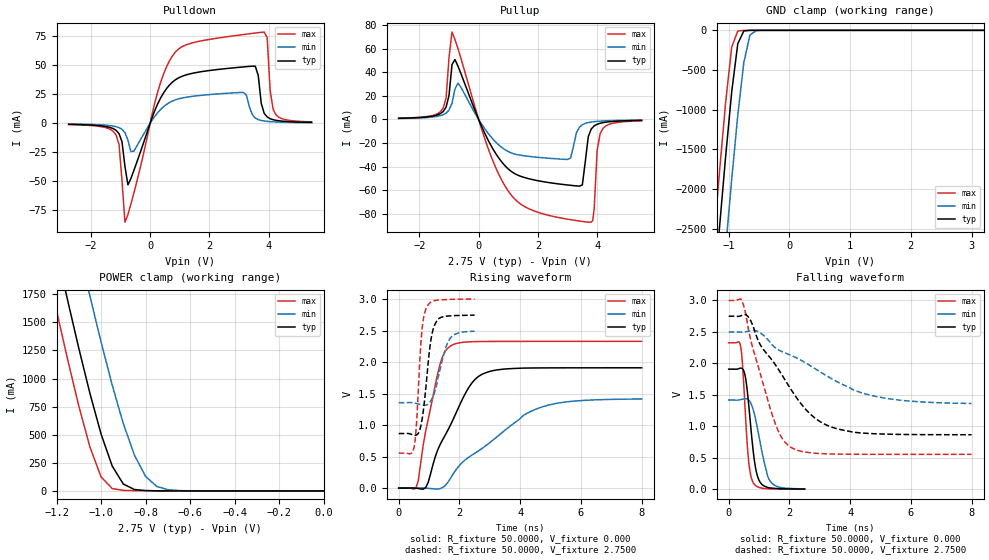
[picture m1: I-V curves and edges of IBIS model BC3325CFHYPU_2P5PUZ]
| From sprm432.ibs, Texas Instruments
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|   Model BC3325CFHYPU_2P5PUZ
[Model]   BC3325CFHYPU_2P5PUZ
Model_type   I/O
Polarity   Non-Inverting
Enable   Active-Low
Vinl =   0.8250V
Vinh =   1.9250V
Vmeas =   1.3750V
Cref =  15.0000pF
Rref = 100.0000M
Vref =  0.000V
C_comp   3.2189pF   3.2468pF   3.2081pF
[Temperature Range]   25.0000   0.1250k   -40.0000
[Voltage Range]   2.7500V   2.5000V   3.0000V
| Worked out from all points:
|   slope of the pulldown table from 0 to 0.412 V, typ, clamps not added: 16.9 ohm
|   slope of the pullup table from 0 to 0.412 V, typ, clamps not added: 18.8 ohm
|   GND clamp passes 1 mA (typ) near -0.66 V on its own axis
|   POWER clamp passes 1 mA (typ) near -0.73 V on its own axis
|   rising waveform, R_fixture 50.0000, V_fixture 0.000: 20-80 % time 1.09ns typ, 2.18ns min, 565ps max; typ from 0.001 V to 1.91 V
|   rising waveform, R_fixture 50.0000, V_fixture 2.7500: 20-80 % time 253ps typ, 352ps min, 179ps max; typ from 0.866 V to 2.74 V
|   falling waveform, R_fixture 50.0000, V_fixture 0.000: 20-80 % time 249ps typ, 370ps min, 182ps max; typ from 1.91 V to 0.003 V
|   falling waveform, R_fixture 50.0000, V_fixture 2.7500: 20-80 % time 1.63ns typ, 2.58ns min, 870ps max; typ from 2.75 V to 0.866 V
[Pulldown]
| voltage   I(typ)   I(min)   I(max)
-2.75V    -942uA     -650uA     -1.139mA
-1.15V    -6.095mA   -2.984mA   -10.11mA
-850mV    -37.32mA   -8.056mA   -85.29mA
-550mV    -40.73mA   -24mA      -60.28mA
350mV     21.58mA    11.77mA    34.97mA
1.05V     40.19mA    21.58mA    65.58mA
3.15V     48.55mA    26.51mA    76.47mA
3.55V     49.14mA    4.498mA    77.79mA
3.85V     8.531mA    1.96mA     78.57mA
3.95V     5.417mA    1.638mA    73.77mA
4.15V     3.05mA     1.228mA    12mA
5.45V     763uA      461uA      1.156mA
[Pullup]
| voltage   I(typ)   I(min)   I(max)
-2.7V     969uA      801uA      1.062mA
-1.2V     6.636mA    4.013mA    9.53mA
-900mV    46.54mA    13.78mA    74.18mA
-700mV    45.39mA    30.78mA    60.33mA
1V        -42.09mA   -27.31mA   -60.87mA
3V        -55.65mA   -33.97mA   -84.69mA
3.4V      -56.64mA   -6.607mA   -86.26mA
3.7V      -14.63mA   -2.671mA   -87.24mA
3.85V     -6.779mA   -2.044mA   -85.88mA
4V        -4.071mA   -1.633mA   -26.15mA
4.1V      -3.234mA   -1.443mA   -12mA
5.5V      -811uA     -542uA     -1.185mA
[GND_clamp]
| voltage   I(typ)   I(min)   I(max)
-2.75V    -17.96A    -19.08A    -17.31A
-1.25V    -3.392A    -4.569A    -2.686A
-1.15V    -2.474A    -3.647A    -1.77A
-1.05V    -1.588A    -2.744A    -906.7mA
-950mV    -773.4mA   -1.875A    -209.9mA
-850mV    -168.6mA   -1.068A    -9.074mA
-750mV    -7.37mA    -403.3mA   -1.005mA
-650mV    -331.2uA   -59.95mA   -203.1uA
-550mV    -99.07uA   -4.004mA   -142.8uA
3.2V      0A         0A         0A
[POWER_clamp]
| voltage   I(typ)   I(min)   I(max)
-2.75V    17.1A      17.93A     16.63A
-1.25V    2.586A     3.492A     2.054A
-1.2V     2.135A     3.04A      1.604A
-1.15V    1.695A     2.594A     1.168A
-1.05V    867.5mA    1.733A     390.4mA
-1V       506.6mA    1.325A     125mA
-950mV    221.5mA    942.3mA    21.02mA
-900mV    61.16mA    598.6mA    4.683mA
-850mV    12.38mA    317.4mA    2.264mA
-800mV    3.105mA    129.1mA    1.319mA
-750mV    1.226mA    39.97mA    719.2uA
0V        226.1pA    1.421nA    243.2pA
[Ramp]
| variable   typ   min   max
dV/dt_r   1.0381/0.9480n   0.3340/0.5367n   1.3934/0.5563n
dV/dt_f   0.8857/1.1637n   0.2933/0.8931n   1.4454/0.8421n
R_load = 50.0000
[Rising Waveform]
R_fixture = 50.0000
V_fixture = 0.000
V_fixture_min = 0.000
V_fixture_max = 0.000
| time   V(typ)   V(min)   V(max)
0s        897uV      859.3uV    954.2uV
565.7ps   -639.9uV   1.934mV    -4.572mV
646.5ps   -5.914mV   1.935mV    121.3mV
888.9ps   8.314mV    -475.1uV   902.6mV
1.293ns   614.7mV    -13.65mV   1.831V
1.697ns   992.8mV    150mV      2.252V
2.424ns   1.675V     527.4mV    2.323V
2.99ns    1.85V      717.4mV    2.327V
4.848ns   1.907V     1.306V     2.328V
8ns       1.909V     1.414V     2.328V
[Rising Waveform]
R_fixture = 50.0000
V_fixture = 2.7500
V_fixture_min = 2.5000
V_fixture_max = 3.0000
| time   V(typ)   V(min)   V(max)
0s        866.2mV    1.355V     555.2mV
505.1ps   839.9mV    1.351V     644.6mV
580.8ps   841mV      1.343V     976.6mV
757.6ps   1.053V     1.321V     2.457V
833.3ps   1.311V     1.315V     2.732V
934.3ps   1.796V     1.323V     2.879V
1.086ns   2.417V     1.407V     2.958V
1.288ns   2.677V     1.735V     2.983V
1.692ns   2.732V     2.373V     2.993V
2.5ns     2.744V     2.488V     2.999V
[Falling Waveform]
R_fixture = 50.0000
V_fixture = 0.000
V_fixture_min = 0.000
V_fixture_max = 0.000
| time   V(typ)   V(min)   V(max)
0s        1.909V     1.417V     2.328V
404ps     1.926V     1.426V     2.244V
454.5ps   1.915V     1.432V     1.991V
530.3ps   1.831V     1.439V     1.376V
631.3ps   1.48V      1.43V      586.2mV
707.1ps   1.098V     1.389V     268.8mV
808.1ps   605.5mV    1.264V     104.5mV
984.8ps   159.3mV    876.3mV    32.88mV
1.364ns   21.51mV    131.5mV    6.622mV
2.5ns     3.408mV    6.945mV    1.603mV
[Falling Waveform]
R_fixture = 50.0000
V_fixture = 2.7500
V_fixture_min = 2.5000
V_fixture_max = 3.0000
| time   V(typ)   V(min)   V(max)
0s        2.75V      2.5V       3V
484.8ps   2.776V     2.499V     2.934V
727.3ps   2.678V     2.519V     2.365V
1.051ns   2.288V     2.482V     1.821V
1.455ns   2.035V     2.283V     1.154V
2.02ns    1.61V      2.135V     676.2mV
2.748ns   1.169V     1.946V     577.2mV
3.556ns   963.5mV    1.714V     559.2mV
5.172ns   876.4mV    1.446V     555.4mV
8ns       866.5mV    1.363V     555.2mV
